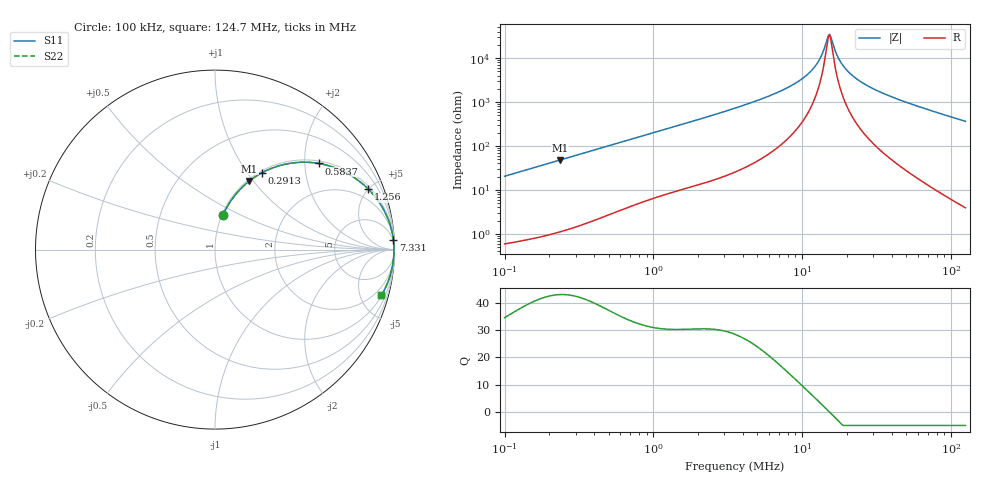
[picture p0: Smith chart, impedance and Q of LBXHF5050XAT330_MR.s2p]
! LBXHF5050XAT330_MR  S-PARAMETER MODEL  ( Standard Model )
! Model Generated by TAIYO YUDEN Corporation (http://www.ty-top.com)
! Version 1.0
! TAIYO YUDEN Control No. 20240926
! Copyright(c) 2024 TAIYO YUDEN CO.,LTD. All Rights Reserved.
! Product Description (link to TY-COMPAS)
! https://ds.yuden.co.jp/TYCOMPAS/or/detail?pn=LBXHF5050XAT330MMR&u=M
! Products Name : Inductors
! Characteristics :
!  Inductance : 33 [uH] , SRF(min) : 12 [MHz] , DC Resistance(max) : 0.276 [Ohm]
!  Rated Current : Saturation  1000 [mA] , Temp Rise  670 [mA] (20 [degC])
!  Case Size : 5.0 x 5.0 / 0.197 x 0.197 [mm/inch] , Thickness : 3.1 / 0.122 [mm/inch]
!  (Conditions: Temperature = 25 [degC] , DC Bias Current = 0 [A])
! External Node Assignments :
!  1  o---GGG---o  2
! GND o---------o GND
! Frequency Range : 0.1MHz  -  124.6553MHz  [ 402 STEP ]
# MHz S RI R 50
! Freq[MHz].  S11 Real  S11 Imag  S21 Real  S21 Imag  S12 Real  S12 Imag  S22 Real  S22 Imag
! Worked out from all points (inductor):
!   401 points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, 100 kHz to 124.7 MHz, reference 50 ohm
!   read as one part in series: L = 32.5 uH near 103.6 kHz
!   highest Q = 43.1 at 235.2 kHz (marker M1), where L = 32.3 uH
!   self-resonance near 14.95 MHz
!   S11 on the Smith chart (normalised r, x): 100 kHz: 1.01, +0.41; 291.3 kHz: 1.03, +1.18; 583.7 kHz: 1.07, +2.35; 1.256 MHz: 1.16, +4.99; 7.331 MHz: 3, +37; 124.7 MHz: 1.08, -7.28
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0.1  0.0453 0.194  0.9547 -0.194  0.9547 -0.194  0.0453 0.194
0.235226  0.1913 0.3819  0.8087 -0.3819  0.8087 -0.3819  0.1913 0.3819
0.291311  0.2634 0.4289  0.7366 -0.4289  0.7366 -0.4289  0.2634 0.4289
0.330013  0.3129 0.4519  0.6871 -0.4519  0.6871 -0.4519  0.3129 0.4519
0.583698  0.5776 0.4801  0.4224 -0.4801  0.4224 -0.4801  0.5776 0.4801
1.089088  0.817 0.3707  0.183 -0.3707  0.183 -0.3707  0.817 0.3707
1.255964  0.8539 0.3371  0.1461 -0.3371  0.1461 -0.3371  0.8539 0.3371
3.530656  0.9768 0.1339  0.0232 -0.1339  0.0232 -0.1339  0.9768 0.1339
7.331042  0.9938 0.0535  0.00615 -0.0535  0.00615 -0.0535  0.9938 0.0535
9.57756  0.9959 0.0322  0.00411 -0.0322  0.00411 -0.0322  0.9959 0.0322
11.65164  0.9967 0.0181  0.0033 -0.0181  0.0033 -0.0181  0.9967 0.0181
13.19963  0.997 0.00951  0.00302 -0.00951  0.00302 -0.00951  0.997 0.00951
14.68918  0.9971 0.00226  0.0029 -0.00226  0.0029 -0.00226  0.9971 0.00226
15.22215  0.9971 -0.00015  0.00289 0.00015  0.00289 0.00015  0.9971 -0.00015
15.77446  0.9971 -0.00256  0.00289 0.00256  0.00289 0.00256  0.9971 -0.00256
16.93993  0.9971 -0.00739  0.00292 0.00739  0.00292 0.00739  0.9971 -0.00739
17.87021  0.997 -0.011  0.00298 0.011  0.00298 0.011  0.997 -0.011
20.60838  0.9967 -0.0209  0.00328 0.0209  0.00328 0.0209  0.9967 -0.0209
26.44805  0.9956 -0.0394  0.00437 0.0394  0.00437 0.0394  0.9956 -0.0394
38.45196  0.992 -0.0718  0.00801 0.0718  0.00801 0.0718  0.992 -0.0718
65.62915  0.9784 -0.1356  0.0216 0.1356  0.0216 0.1356  0.9784 -0.1356
124.6553  0.9274 -0.2542  0.0726 0.2542  0.0726 0.2542  0.9274 -0.2542
